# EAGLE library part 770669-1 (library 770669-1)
Body Features: Connector & Keying Code 1 | Primary Product Color Black | Configuration Features: Number of Rows 3 | PCB Mount Orientation Right Angle | Number of Positions 23 | Contact Features: Contact Mating Area Plating Material Tin | Contact Current Rating (Max) 8 AMP | Contact Type Pin | Housing Features: Centerline (Pitch) 4 MM | Centerline (Pitch) .157 INCH | Industry Standards: UL Flammability Rating UL 94V-0 | Mechanical Attachment: PCB Mount Retention With | PCB Mount Alignment With | Connector Mo Source: Datasheet
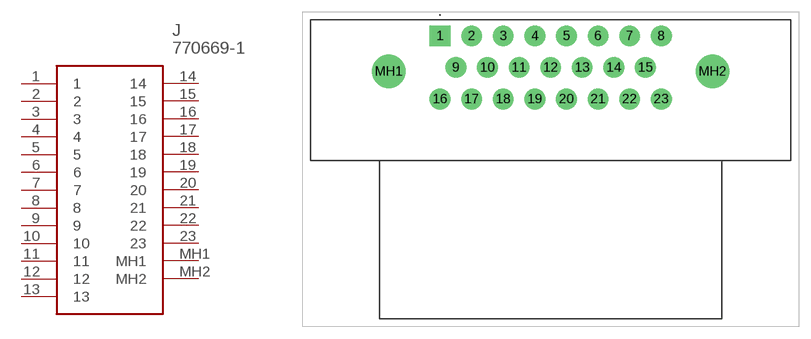
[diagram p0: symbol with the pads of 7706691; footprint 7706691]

Designator prefix J

## 770669-1 (Description: Body Features: Connector & Keying Code 1 | Primary Product Color Black | Configuration Features: Number of Rows 3 | PCB Mount Orientation Right Angle | Number of Positions 23 | Contact Features: Contact Mating Area Plating Material Tin | Contact Current Rating (Max) 8 AMP | Contact Type Pin | Housing Features: Centerline (Pitch) 4 MM | Centerline (Pitch) .157 INCH | Industry Standards: UL Flammability Rating UL 94V-0 | Mechanical Attachment: PCB Mount Retention With | PCB Mount Alignment With | Connector Mo; Height: 32.3mm; Manufacturer_Name: TE Connectivity; Manufacturer_Part_Number: 770669-1; Mouser_Part_Number: 571-770669-1; Mouser_Price-Stock: https://www.mouser.co.uk/ProductDetail/TE-Connectivity/770669-1?qs=bVE8zYB%2Fq2eQrARJAzxzTA%3D%3D)  [7706691]
1  1
2  2
3  3
4  4
5  5
6  6
7  7
8  8
9  9
10  10
11  11
12  12
13  13
14  14
15  15
16  16
17  17
18  18
19  19
20  20
21  21
22  22
23  23
MH1  MH1
MH2  MH2

## Footprint 7706691 (pad centres in mm)
770669-1
drill 1.75 pad 2.625 square: 1 0,0
drill 1.75 pad 2.625: 2 4,0; 3 8,0; 4 12,0; 5 16,0; 6 20,0; 7 24,0; 8 28,0; 9 2,-4; 10 6,-4; 11 10,-4; 12 14,-4; 13 18,-4; 14 22,-4; 15 26,-4; 16 0,-8; 17 4,-8; 18 8,-8; 19 12,-8; 20 16,-8; 21 20,-8; 22 24,-8; 23 28,-8
drill 2.85 pad 4.275: MH1 -6.5,-4.5; MH2 34.5,-4.5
